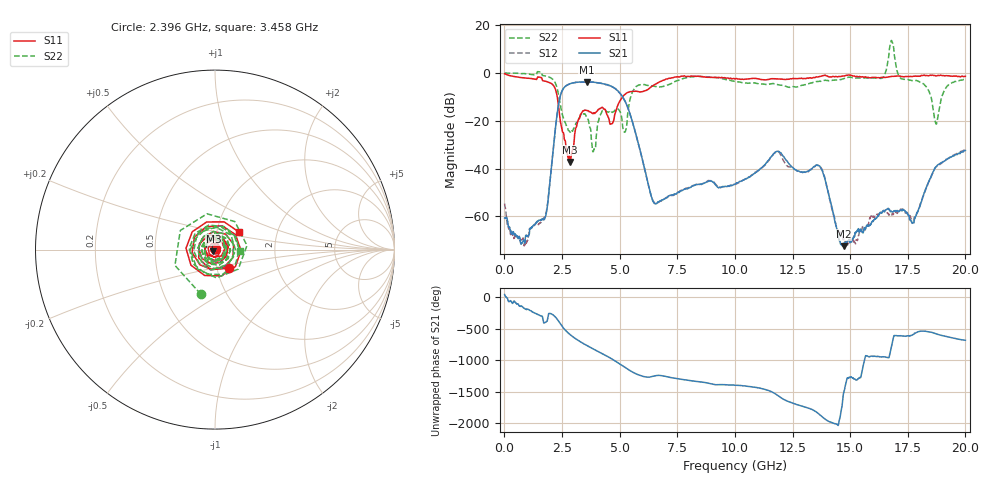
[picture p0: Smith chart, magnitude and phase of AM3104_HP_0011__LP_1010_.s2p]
!Created with skrf (http://scikit-rf.org).
# Hz S RI R 50.0
!freq ReS11 ImS11 ReS21 ImS21 ReS12 ImS12 ReS22 ImS22
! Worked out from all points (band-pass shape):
!   1601 points, 10 MHz to 20 GHz, reference 50 ohm
!   highest |S21| = -3.71 dB at 3.571 GHz (marker M1); lowest = -72.5 dB at 14.72 GHz (marker M2)
!   |S21| within 3 dB of the highest: 2.546 GHz to 4.836 GHz (2.29 GHz wide, 62.1 % of centre)
!   lowest |S11| = -37.2 dB at 2.859 GHz (marker M3), VSWR 1.03, Z = 49.1 - j0.99 ohm
!   |S11| at or under -10 dB: 2.294 GHz to 5.129 GHz (2.835 GHz wide, 76.4 % of centre)
!   |S22| runs from -33.0 to 13.6 dB; largest |S21 - S12| = 0.051
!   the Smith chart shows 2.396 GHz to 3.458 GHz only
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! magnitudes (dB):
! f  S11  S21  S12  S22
! 10 MHz  -0.4  -60.7  -54.7  0.0
! 884.6 MHz  -2.0  -71.2  -71.9  -0.2
! 1.697 GHz  -3.3  -61.5  -60.8  -1.1
! 2.384 GHz  -16.7  -11.4  -11.5  -11.0
! 2.859 GHz  -37.2  -4.5  -4.5  -24.8
! 3.346 GHz  -16.8  -3.8  -3.9  -17.0
! 3.571 GHz  -15.7  -3.7  -3.8  -18.7
! 3.871 GHz  -16.8  -3.9  -3.9  -32.5
! 4.283 GHz  -14.7  -4.5  -4.5  -15.7
! 4.658 GHz  -21.2  -5.6  -5.8  -16.4
! 5.157 GHz  -9.6  -10.4  -10.5  -23.7
! 5.682 GHz  -7.6  -24.8  -24.8  -6.0
! 6.682 GHz  -4.0  -54.1  -54.2  -5.8
! 10.01 GHz  -2.5  -46.6  -46.7  -3.6
! 11.83 GHz  -2.5  -32.9  -32.9  -4.8
! 13.34 GHz  -2.1  -40.1  -40.1  -4.1
! 13.78 GHz  -1.2  -40.7  -40.4  -3.3
! 14.72 GHz  -1.3  -72.5  -69.4  -2.4
! 16.68 GHz  -1.6  -57.2  -59.5  7.2
! 17.74 GHz  -1.4  -62.7  -61.5  -3.1
! 18.73 GHz  -1.2  -39.3  -39.3  -21.3
! 20 GHz  -1.4  -32.5  -32.0  -2.6
